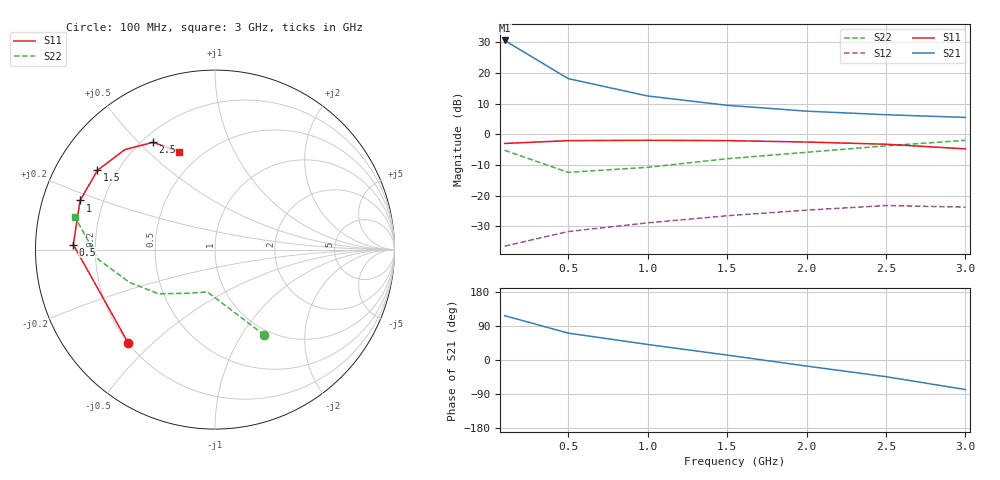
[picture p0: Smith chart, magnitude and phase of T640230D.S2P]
!AT-64023
!S-PARAMETERS at Vce=10V  Ic=70mA.  LAST UPDATED 06-28-94
# ghz s ma r 50
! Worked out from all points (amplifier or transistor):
!   7 points, 100 MHz to 3 GHz, reference 50 ohm
!   highest |S21| = 30.6 dB at 100 MHz (marker M1)
!   |S21| within 3 dB of that: start of sweep to 196.5 MHz
!   unconditionally stable (mu >= 1): nowhere
!   at 500 MHz: K = 0.77, MSG = 24.9 dB, |S12| = -31.7 dB
!   at 1.5 GHz: K = 0.96, MSG = 18.0 dB, |S12| = -26.6 dB
!   at 3 GHz: K = 0.58, MSG = 14.6 dB, |S12| = -23.7 dB
!   S11 on the Smith chart (normalised r, x): 100 MHz: 0.20, -0.42; 500 MHz: 0.12, +0.02; 1 GHz: 0.11, +0.17; 1.5 GHz: 0.13, +0.30; 2.5 GHz: 0.24, +0.55; 3 GHz: 0.38, +0.63
0.1  0.71 -133.0  34.01 117.0  0.015 41.0  0.55 -60.0
0.5  0.79 178.0  8.12 71.0  0.026 33.0  0.24 -100.0
1  0.8 160.0  4.23 41.0  0.036 35.0  0.29 -123.0
1.5  0.79 146.0  2.98 13.0  0.047 31.0  0.4 -142.0
2  0.75 132.0  2.39 -16.0  0.058 21.0  0.51 -159.0
2.5  0.69 120.0  2.09 -44.0  0.069 8.0  0.65 -175.0
3  0.58 110.0  1.89 -78.0  0.065 -16.0  0.8 167.0
